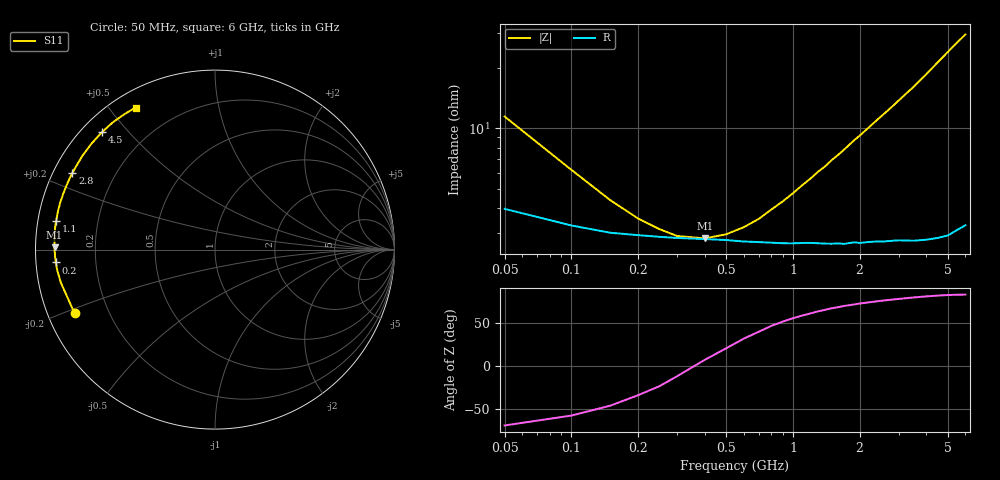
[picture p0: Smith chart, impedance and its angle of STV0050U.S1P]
! SIEMENS Discrete & RF Semiconductors
! BA892
! Si PIN Diode in SCD-80
! IF = 0.05 mA
! S-Parameters:  September  1997
# GHz  S  MA  R  50
!  f  S11
! GHz  MAG  ANG
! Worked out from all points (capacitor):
!   34 points, 50 MHz to 6 GHz, reference 50 ohm
!   read as one part to ground: C = 279 pF near 50 MHz
!   lowest |Z| = 2.82 ohm at 400 MHz (marker M1)
!   series resonance near 363.6 MHz, so ESL is about 690 pH
!   S11 on the Smith chart (normalised r, x): 50 MHz: 0.08, -0.21; 200 MHz: 0.06, -0.04; 1.1 GHz: 0.05, +0.09; 2.8 GHz: 0.05, +0.25; 4.5 GHz: 0.06, +0.42; 6 GHz: 0.07, +0.58
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0.05  0.8592 -155.6
0.1  0.8784 -167.9
0.15  0.8869 -172.7
0.2  0.8895 -175.4
0.25  0.8914 -177.1
0.3  0.8927 -178.6
0.4  0.894 179.2
0.6  0.8969 176.1
0.8  0.8984 173.4
0.9  0.8991 172.2
1.1  0.8991 169.8
1.2  0.8992 168.7
1.3  0.8998 167.5
1.4  0.9004 166.5
1.5  0.9008 165.3
1.6  0.9006 164.3
1.7  0.9015 163.2
1.9  0.9003 161.0
2  0.9013 160.0
2.4  0.901 155.8
2.8  0.9018 151.8
3  0.9022 149.7
3.5  0.9049 144.7
4  0.9067 139.4
4.5  0.9082 134.0
5  0.9094 128.8
5.5  0.9077 123.8
6  0.9068 119.2
